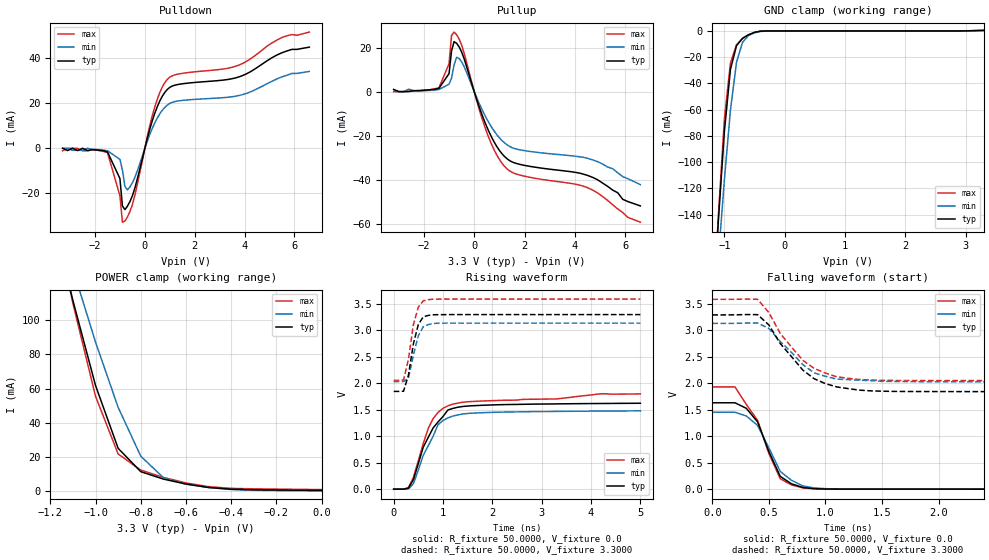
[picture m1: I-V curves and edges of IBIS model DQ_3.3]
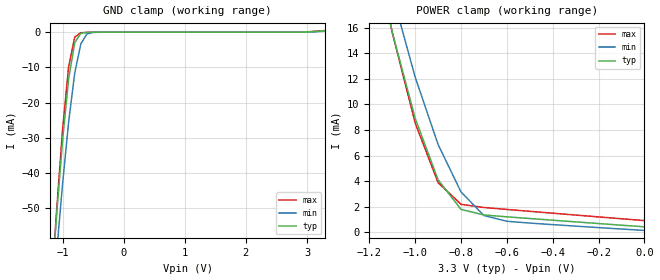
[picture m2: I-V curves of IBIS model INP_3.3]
|*** ISSI Synchronous Sram IBIS Model ***
[IBIS ver]	3.2
[File name]	is61lf204836b119bga.ibs
[File Rev]	1.0
[Date]	May 13,2013
[Notes]
|--- Version History --------------------------------
|1.0: prelimiary
[Disclaimer]	This information is for modeling purpose only
		and is not guaranteed
[Copyright]	INTEGRATED SILICON SOLUTION, INC. 2011
[Component]	IS61LF204836B_119BGA
[Manufacturer]	ISSI
[Package]
| variable   typ   min   max
R_pkg		100.34m			23.84m			218.59m
L_pkg		1.3400nH		0.3700nH		3.0300nH
C_pkg		41.410pF		0.4200pF		150.38pF
[Pin]  signal_name   model_name   R_pin   L_pin   C_pin
U7   VDDQ   POWER
U6   NC   NC
U5   TDO   DQ_3.3
U4   TCK   INP_3.3
U3   TDI   INP_3.3
U2   TMS   INP_3.3
U1   VDDQ   POWER
T7   ZZ   INP_3.3
T6   A   INP_3.3
T5   A   INP_3.3
T4   A   INP_3.3
T3   A   INP_3.3
T2   A   INP_3.3
T1   NC   NC
R7   NC   NC
R6   A   INP_3.3
R5   NC   NC
R4   VDD   POWER
R3   MODE   INP_3.3
R2   A   INP_3.3
R1   NC   NC
P7   DQa   DQ_3.3
P6   DQPa   DQ_3.3
P5   VSS   GND
P4   A0   INP_3.3
P3   VSS   GND
P2   DQPd   DQ_3.3
P1   DQd   DQ_3.3
N7   DQa   DQ_3.3
N6   DQa   DQ_3.3
N5   VSS   GND
N4   A1   INP_3.3
N3   VSS   GND
N2   DQd   DQ_3.3
N1   DQd   DQ_3.3
M7   VDDQ   POWER
M6   DQa   DQ_3.3
M5   VSS   GND
M4   BWEB   INP_3.3
M3   VSS   GND
M2   DQd   DQ_3.3
M1   VDDQ   POWER
L7   DQa   DQ_3.3
L6   DQa   DQ_3.3
L5   BWaB   INP_3.3
L4   NC   NC
L3   BWdB   INP_3.3
L2   DQd   DQ_3.3
L1   DQd   DQ_3.3
K7   DQa   DQ_3.3
K6   DQa   DQ_3.3
K5   VSS   GND
K4   CLK   INP_3.3
K3   VSS   GND
K2   DQd   DQ_3.3
K1   DQd   DQ_3.3
J7   VDDQ   POWER
J6   VDD   POWER
J5   NC   NC
J4   VDD   POWER
J3   NC   NC
J2   VDD   POWER
J1   VDDQ   POWER
H7   DQb   DQ_3.3
H6   DQb   DQ_3.3
H5   VSS   GND
H4   GWB   INP_3.3
H3   VSS   GND
H2   DQc   DQ_3.3
H1   DQc   DQ_3.3
G7   DQb   DQ_3.3
G6   DQb   DQ_3.3
G5   BWbB   INP_3.3
G4   ADVB   INP_3.3
G3   BWcB   INP_3.3
G2   DQc   DQ_3.3
G1   DQc   DQ_3.3
F7   VDDQ   POWER
F6   DQb   DQ_3.3
F5   VSS   GND
F4   OEB   INP_3.3
F3   VSS   GND
F2   DQc   DQ_3.3
F1   VDDQ   POWER
E7   DQb   DQ_3.3
E6   DQb   DQ_3.3
E5   VSS   GND
E4   CEB   INP_3.3
E3   VSS   GND
E2   DQc   DQ_3.3
E1   DQc   DQ_3.3
D7   DQb   DQ_3.3
D6   DQPb   DQ_3.3
D5   VSS   GND
D4   NC   NC
D3   VSS   GND
D2   DQPc   DQ_3.3
D1   DQc   DQ_3.3
C7   NC   Nc
C6   A   INP_3.3
C5   A   INP_3.3
C4   VDD   POWER
C3   A   INP_3.3
C2   A   INP_3.3
C1   NC   NC
B7   NC   NC
B6   A   INP_3.3
B5   A   INP_3.3
B4   ADSCB   INP_3.3
B3   A   INP_3.3
B2   A   INP_3.3
B1   NC   NC
A7   VDDQ   POWER
A6   A   INP_3.3
A5   A   INP_3.3
A4   ADSPB   INP_3.3
A3   A   INP_3.3
A2   A   INP_3.3
A1   VDDQ   POWER
| Models and submodels in the file (2): DQ_3.3 (3-state), INP_3.3 (Input)
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|   Model DQ_3.3
[Model]		DQ_3.3
Model_type	3-state
Polarity   Non-Inverting
Enable   Active-Low
Vmeas = 	0.7500V
Cref = 		5.0000pF
Rref = 		50.0000
Vref = 		1.2500V
C_comp   3.8290pF   3.3420pF   4.0300pF|
[Temperature Range]	  25.0000   100.0000   0.0
[Voltage Range]   3.3000V   3.1350V   3.6000V
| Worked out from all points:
|   slope of the pulldown table from 0 to 0.495 V, typ, clamps not added: 26.9 ohm
|   slope of the pullup table from 0 to 0.495 V, typ, clamps not added: 31.2 ohm
|   GND clamp passes 1 mA (typ) near -0.49 V on its own axis
|   POWER clamp passes 1 mA (typ) near -0.36 V on its own axis
|   rising waveform, R_fixture 50.0000, V_fixture 0.0: 20-80 % time 480ps typ, 408ps min, 447ps max; typ from 0 V to 1.62 V
|   rising waveform, R_fixture 50.0000, V_fixture 3.3000: 20-80 % time 178ps typ, 175ps min, 176ps max; typ from 1.84 V to 3.29 V
|   falling waveform, R_fixture 50.0000, V_fixture 0.0: 20-80 % time 195ps typ, 217ps min, 242ps max; typ from 1.63 V to 0 V
|   falling waveform, R_fixture 50.0000, V_fixture 3.3000: 20-80 % time 343ps typ, 315ps min, 335ps max; typ from 3.29 V to 1.84 V
[Pulldown]
|Voltage	  I(typ)   I(min)   I(max)
-3.3V     0A         0A         -1.1mA
-1.5V     -1.6mA     -1.08mA    -1.87mA
-1V       -13.48mA   -4.95mA    -21.15mA
-900mV    -25.69mA   -9.639mA   -32.88mA
-800mV    -27.28mA   -16.91mA   -32.39mA
-700mV    -25.77mA   -18.5mA    -30.54mA
-500mV    -21.13mA   -15.36mA   -25.04mA
400mV     15.63mA    11.35mA    18.49mA
900mV     26.18mA    19.21mA    30.66mA
3.7V      31.51mA    23.31mA    36.7mA
5.5V      42.5mA     31.77mA    49.28mA
6.6V      45mA       34.2mA     51.7mA
[Pullup]
|Voltage	  I(typ)   I(min)   I(max)
-3.2V     1mA        900uA      0A
-1.4V     1.5mA      990uA      1.76mA
-1V       8.19mA     3.366mA    12.71mA
-900mV    18.53mA    6.147mA    25.54mA
-800mV    22.75mA    12.11mA    27.08mA
-700mV    21.98mA    15.63mA    25.89mA
-500mV    18.06mA    13.53mA    21.17mA
400mV     -13.22mA   -10.27mA   -15.35mA
1.2V      -29.47mA   -23.28mA   -33.95mA
1.9V      -33.32mA   -26.66mA   -38.21mA
4.5V      -38.1mA    -30.33mA   -43.68mA
6.6V      -52mA      -42.3mA    -59.4mA
[GND_clamp]
|Voltage	  I(typ)   I(min)   I(max)
-3.3V     -1.893A    -1.626A    -2.116A
-1.2V     -220.2mA   -237.3mA   -225.5mA
-1.1V     -144.4mA   -173.5mA   -140.5mA
-1V       -76.37mA   -113.2mA   -66.76mA
-900mV    -29.2mA    -60.35mA   -24.24mA
-800mV    -11.34mA   -23.99mA   -10.52mA
-700mV    -5.573mA   -8.7mA     -5.892mA
-600mV    -2.907mA   -3.457mA   -3.011mA
-500mV    -1.075mA   -1.407mA   -999.8uA
-300mV    -9.492uA   -41.34uA   -5.052uA
3.3V      423.1uA    322.6uA    488.5uA
[POWER_clamp]
|Voltage	  I(typ)   I(min)   I(max)
-3.3V     1.424A     1.197A     1.604A
-1.2V     166.3mA    175.1mA    171.7mA
-1.1V     111.5mA    129.9mA    109.8mA
-1V       61.82mA    87.17mA    55.51mA
-900mV    25.05mA    49.03mA    21.74mA
-800mV    11.41mA    20.46mA    12.33mA
-700mV    7.064mA    7.924mA    8.056mA
-600mV    4.166mA    4.141mA    4.82mA
-500mV    2.143mA    2.162mA    2.625mA
-400mV    1.124mA    995.4uA    1.625mA
0V        423.1uA    141.8uA    910.6uA
[Ramp]
| variable   typ   min   max
dV/dt_r		0.9120/0.3809n   0.7302/0.3836n   1.1604/0.3404n
dV/dt_f		0.8694/0.3076n   0.7542/0.2869n   0.9210/0.3315n
R_load =	50.0000
[Rising Waveform]
R_fixture=	50.0000
V_fixture=	0.0
V_fixture_min=	0.0
V_fixture_max=	0.0
|time   V(typ)   V(min)   V(max)
0s        0V         533.2nV    0V
300ps     18.56mV    3.797mV    30.05mV
400ps     179mV      102.4mV    219.2mV
600ps     791.3mV    638.4mV    860.4mV
700ps     973.8mV    816.1mV    1.144V
900ps     1.268V     1.216V     1.448V
1.1ns     1.494V     1.344V     1.571V
1.4ns     1.559V     1.419V     1.639V
1.9ns     1.585V     1.445V     1.665V
5ns       1.62V      1.476V     1.797V
[Rising Waveform]
R_fixture=	50.0000
V_fixture=	3.3000
V_fixture_min=	3.1350
V_fixture_max=	3.6000
|time   V(typ)   V(min)   V(max)
0s        1.843V     2.029V     2.051V
200ps     1.847V     2.03V      2.057V
300ps     2.15V      2.093V     2.449V
400ps     2.742V     2.529V     3.102V
500ps     3.104V     2.892V     3.434V
600ps     3.25V      3.063V     3.552V
700ps     3.276V     3.103V     3.573V
800ps     3.288V     3.123V     3.583V
1ns       3.291V     3.131V     3.585V
5ns       3.292V     3.131V     3.585V
[Falling Waveform]
R_fixture=	50.0000
V_fixture=	0.0
V_fixture_min=	0.0
V_fixture_max=	0.0
|time   V(typ)   V(min)   V(max)
0s        1.632V     1.453V     1.932V
200ps     1.632V     1.452V     1.931V
300ps     1.527V     1.382V     1.602V
400ps     1.271V     1.204V     1.299V
500ps     710mV      779.4mV    671.9mV
600ps     241.6mV    335.5mV    197.9mV
700ps     100.8mV    166.6mV    80.02mV
800ps     32.06mV    61.86mV    23.86mV
1.2ns     262.2uV    1.546mV    276.4uV
5ns       29.31uV    38.72uV    18.07uV
[Falling Waveform]
R_fixture=	50.0000
V_fixture=	3.3000
V_fixture_min=	3.1350
V_fixture_max=	3.6000
|time   V(typ)   V(min)   V(max)
0s        3.292V     3.132V     3.586V
400ps     3.297V     3.139V     3.587V
500ps     3.102V     3.036V     3.335V
600ps     2.752V     2.791V     2.944V
800ps     2.249V     2.353V     2.434V
900ps     2.087V     2.196V     2.281V
1.1ns     1.931V     2.079V     2.123V
1.3ns     1.871V     2.058V     2.072V
1.6ns     1.847V     2.035V     2.054V
5ns       1.843V     2.029V     2.051V
|   Model INP_3.3
[Model]		INP_3.3
Model_type	Input
Polarity   Non-Inverting
Enable   Active-Low
Vinl = 		0.8000V
Vinh = 		2.0000V
C_comp   3.8290pF   3.3420pF   4.0300pF|
[Temperature Range]	  25.0000   100.0000   0.0
[Voltage Range]   3.3000V   3.1350V   3.6000V
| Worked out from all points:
|   GND clamp passes 1 mA (typ) near -0.73 V on its own axis
|   POWER clamp passes 1 mA (typ) near -0.45 V on its own axis
[GND_clamp]
|Voltage	  I(typ)   I(min)   I(max)
-3.3V     -664.2mA   -601mA     -729.6mA
-1.2V     -76.89mA   -84.89mA   -78.19mA
-1.1V     -52.83mA   -63.46mA   -51.66mA
-1V       -30.98mA   -43.42mA   -27.92mA
-900mV    -13.28mA   -25.61mA   -9.811mA
-800mV    -2.971mA   -11.61mA   -1.401mA
-700mV    -287uA     -3.303mA   -148.3uA
-600mV    -52.18uA   -480.7uA   -48.72uA
-500mV    -11.21uA   -45.78uA   -9.079uA
2.8V      415nA      176.2nA    769.3nA
3.3V      423.1uA    321.5uA    488.5uA
[POWER_clamp]
|Voltage	  I(typ)   I(min)   I(max)
-3.3V     318.3mA    284.6mA    350.6mA
-1.2V     23.85mA    26.22mA    24.49mA
-1.1V     15.64mA    18.66mA    15.62mA
-1V       8.908mA    12.13mA    8.545mA
-900mV    4.097mA    6.862mA    3.88mA
-800mV    1.786mA    3.15mA     2.181mA
-700mV    1.348mA    1.305mA    1.934mA
-600mV    1.205mA    856uA      1.783mA
0V        423.1uA    141.8uA    910.6uA
